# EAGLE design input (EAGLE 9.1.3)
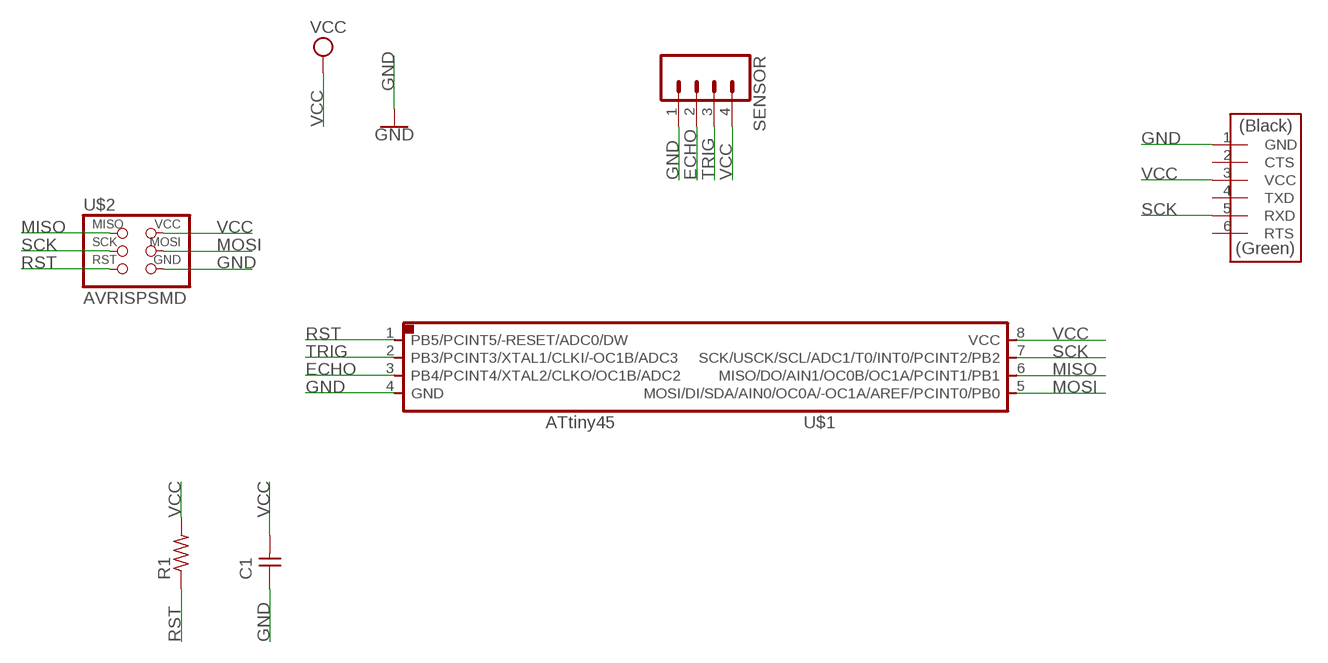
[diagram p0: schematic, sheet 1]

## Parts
C1  CAP-UNPOLARIZEDFAB  [C1206FAB]
FTDI  FTDI-SMD-HEADER  [1X06SMD]
R1  RES-US1206FAB  [R1206FAB]
SENSOR  CONN_04  [1X04]
U$1  ATTINY45SI  [SOIC8]
U$2  AVRISPSMD  [2X03SMD]

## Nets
ECHO: SENSOR.2 U$1.3(PB4/PCINT4/XTAL2/CLKO/OC1B/ADC2)
GND: C1.1 FTDI.1(GND) SENSOR.1 U$1.4(GND) U$2.6(GND)
MISO: U$1.6(MISO/DO/AIN1/OC0B/OC1A/PCINT1/PB1) U$2.1(MISO)
MOSI: U$1.5(MOSI/DI/SDA/AIN0/OC0A/-OC1A/AREF/PCINT0/PB0) U$2.4(MOSI)
RST: R1.1 U$1.1(PB5/PCINT5/-RESET/ADC0/DW) U$2.5(RST)
SCK: FTDI.5(RXD) U$1.7(SCK/USCK/SCL/ADC1/T0/INT0/PCINT2/PB2) U$2.3(SCK)
TRIG: SENSOR.3 U$1.2(PB3/PCINT3/XTAL1/CLKI/-OC1B/ADC3)
VCC: C1.2 FTDI.3(VCC) R1.2 SENSOR.4 U$1.8(VCC) U$2.2(VCC)
Unconnected: FTDI.2(CTS) FTDI.4(TXD) FTDI.6(RTS)

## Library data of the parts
C1 = fab:CAP-UNPOLARIZED
FTDI = fab:FTDI-SMD-HEADER
R1 = fab:RES-US: Resistor (US Symbol)
SENSOR = SparkFun-Connectors:CONN_04: Multi connection point. Often used as Generic Header-pin footprint for 0.1 inch spaced/style header connections On any of the 0.1 inch spaced packages, you can populate with these: Break Away Headers - Straight (PRT-00116) Break Away Male Headers - Right Angle (PRT-00553) Female Headers (PRT-00115)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; PROD_ID: CONN-09696
U$1 = fab:ATTINY45
U$2 = fab:AVRISP

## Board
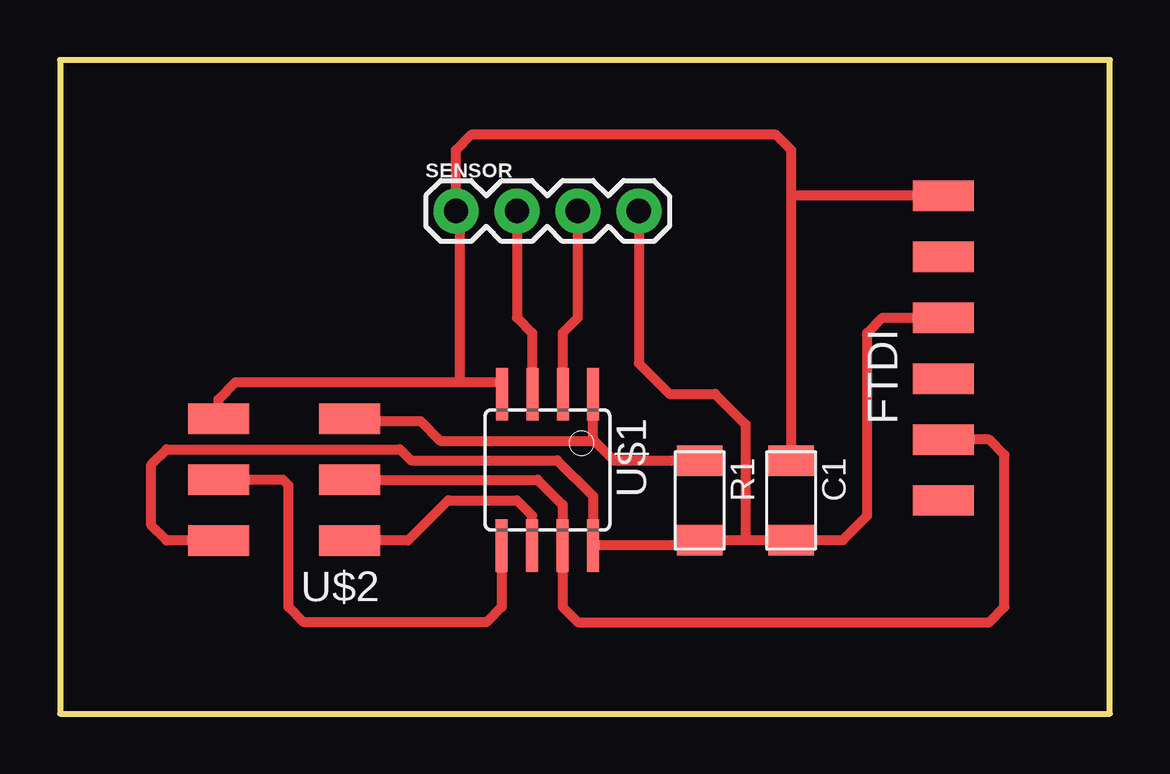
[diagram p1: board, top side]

Size 43.77 x 27.25 mm. Coordinates in mm from the lower left corner, seen from the top.
Outline: 0,0 43.77,0 43.77,27.25 0,27.25 0,0
Copper layers (1*16): Top 0.035mm / dielectric 1.5mm / Bottom 0.035mm
Design rules "fabcity-designrules": minimum track width 10mil, minimum drill 32mil, track to track 16mil, track to pad 16mil, pad to pad 16mil, via to via 16mil, smd to smd 6mil, copper to edge 16mil, drill to drill 16mil, minimum pad ring 10mil, minimum via ring 8mil, stop-mask expansion 4mil, vias tented up to drill 0mil, thermal gap 16mil

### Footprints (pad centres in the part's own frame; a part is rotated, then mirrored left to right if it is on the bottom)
C1206FAB = smd 1.27 x 1.905: 1 -1.651,0; 2 1.651,0
1X06SMD = smd 2.54 x 1.27: 1 0,6.35; 2 0,3.81; 3 0,1.27; 4 0,-1.27; 5 0,-3.81; 6 0,-6.35
R1206FAB = smd 1.27 x 1.905: 1 -1.651,0; 2 1.651,0
1X04 = drill 1.016 pad 1.88: 1 0,0; 2 2.54,0; 3 5.08,0; 4 7.62,0
SOIC8 = smd 0.5 x 2.2: 1 -1.905,-3.154; 2 -0.645,-3.154; 3 0.625,-3.154; 4 1.895,-3.154; 5 1.905,3.154; 6 0.635,3.154; 7 -0.635,3.154; 8 -1.905,3.154
2X03SMD = smd 2.54 x 1.27: 1 -2.54,2.54; 2 2.92,2.54; 3 -2.54,0; 4 2.92,0; 5 -2.54,-2.54; 6 2.92,-2.54

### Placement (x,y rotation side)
C1  30.48,8.89 270 top
FTDI  36.83,15.24 0 top
R1  26.67,8.89 270 top
SENSOR  16.51,20.95 0 top
U$1  20.32,10.16 180 top
U$2  9.53,9.75 180 top

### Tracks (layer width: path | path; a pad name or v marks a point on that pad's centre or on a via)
ECHO
  Top 0.406: SENSOR.2 19.05,16.51 19.68,15.88 19.68,13.32 U$1.3
GND
  Top 0.406: C1.1 30.48,21.59 | 30.48,21.59 30.48,23.5 29.84,24.13 17.14,24.13 16.51,23.5 SENSOR.1 16.66,20.8 16.66,13.82 | FTDI.1 30.48,21.59 | U$2.6 6.61,13.11 7.32,13.82 16.66,13.82 | 16.66,13.82 18.29,13.82 18.43,13.68 U$1.4
MISO
  Top 0.406: U$1.6 19.68,8.26 19.05,8.89 16.18,8.89 14.5,7.21 U$2.1
MOSI
  Top 0.406: U$1.5 18.41,4.45 17.78,3.81 10.16,3.81 9.53,4.45 9.53,9.53 9.3,9.75 U$2.4
RST
  Top 0.406: R1.1 23.11,10.54 22.23,11.43 | 22.23,11.43 U$1.1 | U$2.5 12.17,12.19 15.04,12.19 15.85,11.38 22.17,11.38 22.23,11.43
SCK
  Top 0.406: FTDI.5 38.73,11.43 39.37,10.79 39.37,4.45 38.73,3.81 21.59,3.81 20.95,4.45 20.95,6.99 U$1.7 20.95,8.71 19.91,9.75 U$2.3
TRIG
  Top 0.406: U$1.2 20.96,15.88 21.59,16.51 SENSOR.3
VCC
  Top 0.406: 28.57,7.24 R1.2 26.44,7.01 U$1.8 22.23,9.07 20.73,10.57 14.63,10.57 14.17,11.02 4.45,11.02 3.81,10.39 3.81,7.85 4.45,7.21 U$2.2 | 28.57,7.24 C1.2 32.64,7.24 33.66,8.26 33.66,15.88 34.29,16.51 FTDI.3 | SENSOR.4 24.13,14.61 25.4,13.34 27.3,13.34 28.57,12.06 28.57,7.24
